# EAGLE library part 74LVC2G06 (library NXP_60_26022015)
Inverters with open-drain outputs The 74LVC2G06 provides two inverting buffers. The output of this device is an open drain and can be connected to other open-drain outputs to implement active-LOW wired-OR or active-HIGH wired-AND functions. Input can be driven from either 3.3 V or 5 V devices. This feature allows the use of this device in a mixed 3.3 V and 5 V environment. Schmitt trigger action at all inputs makes the circuit tolerant for slower input rise and fall time. This device is fully specified for partial power-down applications using IOFF. The IOFF circuitry disables the output, preventing the damaging backflow current through the device when it is powered down. AAL Eindhoven MK
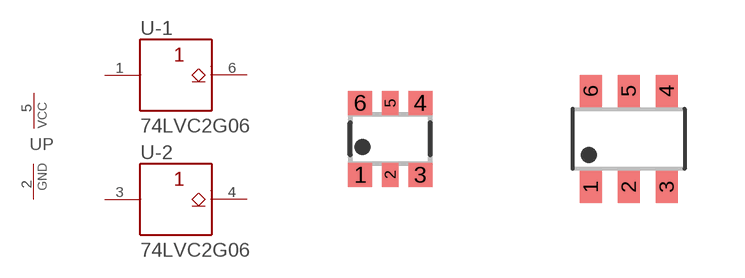
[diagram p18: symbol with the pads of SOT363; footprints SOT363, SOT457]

Designator prefix U; gates P=PWRN -1=BUFFER_OPENDRAIN -2=BUFFER_OPENDRAIN

## 74LVC2G06GW (12NC: 9352 738 82125)  [SOT363]
1  -1:A  in
2  P:GND  pwr
3  -2:A  in
4  -2:Y  oc
5  P:VCC  pwr
6  -1:Y  oc

## 74LVC2G06GV (12NC: 9352 738 81125)  [SOT457]
Pads as for SOT363

## 74LVC2G06GM (12NC: 9352 771 68132)  [SOT886]
Pads as for SOT363

## 74LVC2G06GF (12NC: 9352 824 31132)  [SOT891]
Pads as for SOT363

## 74LVC2G06GS (12NC: 9352 929 27132)  [SOT1202]
Pads as for SOT363

## 74LVC2G06GN (12NC: 9352 917 99132)  [SOT1115]
Pads as for SOT363

## Footprint SOT363 (pad centres in mm)
SOT363 Plastic surface-mounted package; 6 leads JEDEC: -- IEC: -- JEITA: SC-88
smd 0.6 x 0.6: 1 -0.75,-0.9; 3 0.75,-0.9; 4 0.75,0.9; 6 -0.75,0.9
smd 0.4 x 0.6: 2 0,-0.9; 5 0,0.9

## Footprint SOT457 (pad centres in mm)
SOT457 TSOP6: Plastic surface-mounted package; 6 lead JEIDA: SC73 A.K.A. SOT23-6
smd 0.55 x 0.8: 1 -0.95,-1.2; 2 0,-1.2; 3 0.95,-1.2; 4 0.95,1.2; 5 0,1.2; 6 -0.95,1.2

## Footprint SOT886 (pad centres in mm)
SOT886 XSON6: plastic extremely thin small outline package; no leads; 6 terminals; body 1 x 1.45 x 0.5 mm JEDEC: MO-252 IEC: ---
smd 0.27 x 0.325: 1 -0.5,-0.338; 2 0,-0.338; 3 0.5,-0.338; 4 0.5,0.338; 5 0,0.338; 6 -0.5,0.338

## Footprint SOT891 (pad centres in mm)
SOT891 XSON6: plastic extremely thin small outline package; no leads; 6 terminals; body 1 x 1 x 0.5 mm JEDEC: -- IEC: ---
smd 0.15 x 0.5: 1 -0.35,-0.35; 2 0,-0.35; 3 0.35,-0.35; 4 0.35,0.35; 5 0,0.35; 6 -0.35,0.35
